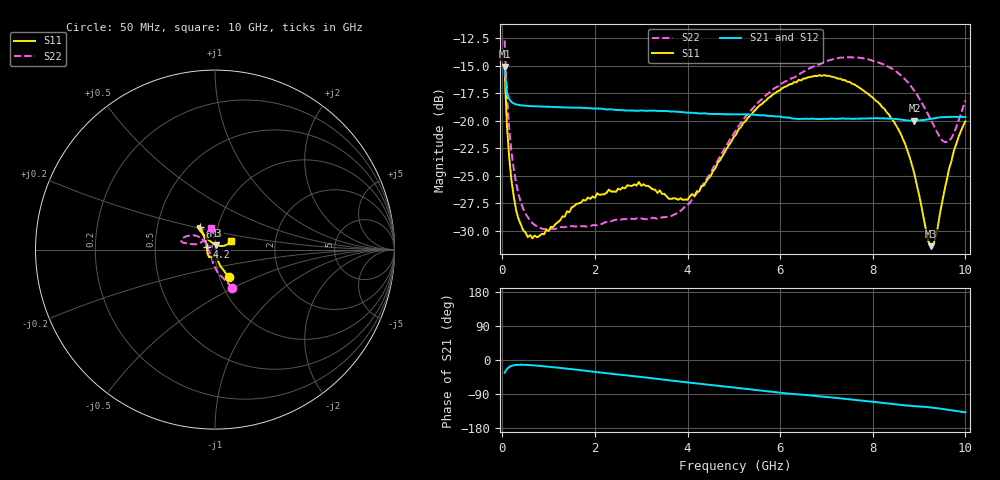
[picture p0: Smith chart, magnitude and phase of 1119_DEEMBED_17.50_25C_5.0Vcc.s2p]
!Hittite Microwave Corp.
!Digital Attenuator/PhaseShifter Rev 1.4.0
!Filename: C:\DATA\DATA\1119_DEEMBED_17.50_25C_5.0Vcc.s2p
!VNA ID: Agilent Technologies,N5224A,MY51441122,A.10.45.03
!Device type:
!2 Port Calibration.
!Temp(C): 25
!Lot Number:
!Serial Number:
!Operator:
!Misc:
!Attenuator:  17.500
# GHZ S DB R 50.0
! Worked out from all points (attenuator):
!   200 points, 50 MHz to 10 GHz, reference 50 ohm
!   highest |S21| = -15.08 dB at 50 MHz (marker M1); lowest = -20.0 dB at 8.9 GHz (marker M2)
!   lowest |S11| = -31.4 dB at 9.25 GHz (marker M3), VSWR 1.06, Z = 50.6 + j2.63 ohm
!   |S11| at or under -10 dB: start of sweep to end of sweep
!   |S22| runs from -29.9 to -12.7 dB; largest |S21 - S12| = 0.00039
!   S11 on the Smith chart (normalised r, x): 50 MHz: 1.11, -0.35; 4.2 GHz: 0.91, +0.02; 6.4 GHz: 0.82, +0.22; 10 GHz: 1.19, +0.11
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0.05  -15.34 -63.4  -15.08 -33.4  -15.08 -33.4  -12.68 -65.5
0.1  -20.39 -72.2  -17.39 -23.8  -17.39 -23.8  -17.62 -82.8
0.2  -25.51 -75.6  -18.30 -15.5  -18.31 -15.5  -22.91 -99.6
0.3  -28.18 -76.0  -18.51 -13.1  -18.51 -13.1  -25.71 -109.4
0.45  -29.96 -76.0  -18.61 -12.6  -18.61 -12.6  -28.00 -119.9
0.9  -30.34 -87.4  -18.71 -16.5  -18.71 -16.5  -29.86 -133.9
1.75  -27.20 -111.1  -18.82 -27.8  -18.82 -27.8  -29.60 -138.3
2.95  -25.58 -130.5  -19.07 -44.0  -19.07 -44.1  -28.91 -157.4
3.4  -26.34 -148.9  -19.10 -50.5  -19.10 -50.5  -28.85 -170.6
3.8  -27.19 -170.7  -19.18 -56.4  -19.19 -56.5  -28.37 173.6
4.2  -26.42 164.2  -19.31 -61.9  -19.32 -61.9  -26.59 156.8
5.05  -21.25 131.6  -19.39 -73.0  -19.41 -73.0  -20.83 140.3
5.55  -18.61 125.5  -19.50 -80.1  -19.50 -80.1  -18.22 142.6
6.4  -16.26 123.5  -19.83 -90.8  -19.85 -90.8  -15.81 151.1
6.7  -15.96 124.6  -19.81 -94.1  -19.82 -94.1  -15.08 154.9
7.5  -16.46 127.9  -19.80 -103.8  -19.81 -103.9  -14.21 164.0
8.35  -19.43 127.8  -19.80 -115.1  -19.80 -115.1  -15.10 167.6
8.9  -24.84 121.0  -19.99 -121.5  -19.99 -121.6  -17.27 166.7
9.25  -31.42 75.4  -19.83 -125.2  -19.84 -125.3  -19.89 161.2
9.35  -30.70 49.0  -19.75 -126.6  -19.77 -126.7  -20.71 156.1
9.65  -24.34 22.5  -19.65 -131.8  -19.66 -131.8  -21.82 126.7
10  -20.04 28.1  -19.66 -138.1  -19.66 -138.1  -18.14 99.5
